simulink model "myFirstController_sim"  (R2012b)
settings: Solver=ode45  StartTime=0.0  StopTime=15  RelTol=1e-3
undefined symbols (not defined in the file): A, B, C_all

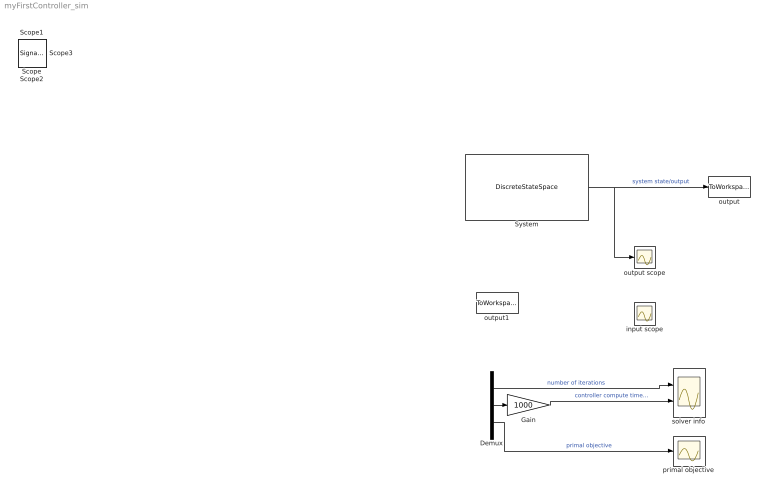
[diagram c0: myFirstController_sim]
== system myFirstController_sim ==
  Demux : Demux  Outputs=3
  Gain : Gain  Gain=1000
  System : DiscreteStateSpace  A=A  B=B  C=C_all  D=zeros(2,1)  X0=[0; 6]
  input scope : Scope
  output : ToWorkspace  VariableName=simulink_res  SampleTime=-1  SaveFormat=Timeseries
  output scope : Scope
  output1 : ToWorkspace  VariableName=solverinfo  SampleTime=-1  SaveFormat=Timeseries
  primal objective : Scope
  solver info : Scope  NumInputPorts=2
  Scope : SignalViewerScope  IOType=viewer  ZoomMode=yonly  RefreshTime=0.035000
  Scope1 : SignalViewerScope  IOType=viewer  RefreshTime=0.035000
  Scope2 : SignalViewerScope  IOType=viewer  RefreshTime=0.035000
  Scope3 : SignalViewerScope  IOType=viewer  RefreshTime=0.035000
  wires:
  System/1 -> output scope/1, output/1  "system state/output"
  ? -> input scope/1, System/1  "optimal input"
  ? -> Demux/1, output1/1  "solver info"
  Demux/2 -> Gain/1
  Gain/1 -> solver info/2  "controller compute time in ms"
  Demux/1 -> solver info/1  "number of iterations"
  Demux/3 -> primal objective/1  "primal objective"
